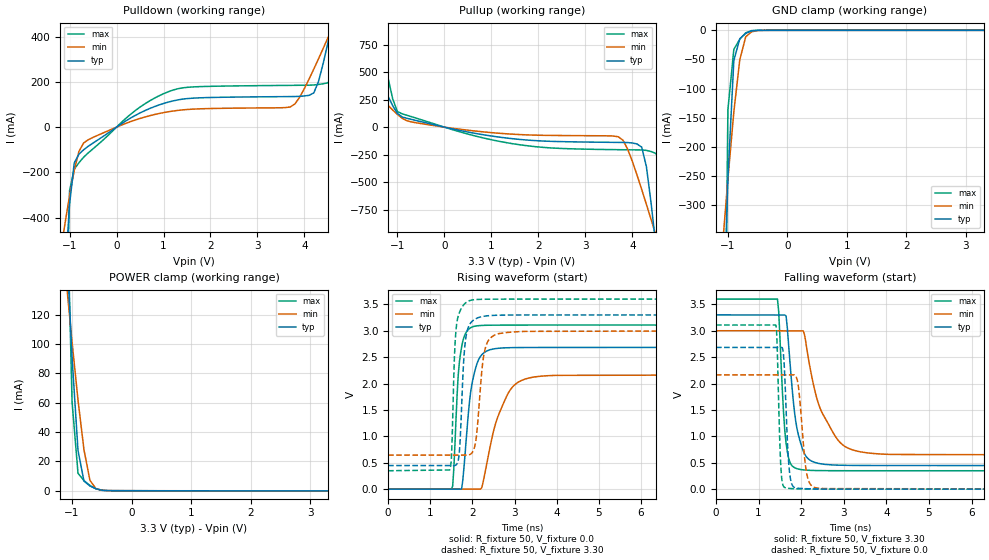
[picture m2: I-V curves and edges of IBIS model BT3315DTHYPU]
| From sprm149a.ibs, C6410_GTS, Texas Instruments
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[Model]   BT3315DTHYPU
Model_type   I/O
Vinh = 2.00
Vinl = 0.80
Enable   Active-Low
Polarity   Non-Inverting
| signals   A, GZ, Y
Vmeas = 1.5
|   typ   min   max
C_comp   1.5797p   1.5046p   1.7659p
|   typ   min   max
[Temperature Range]   25   -40   125
|   typ   min   max
[Voltage Range]   3.30V   3.00V   3.60V
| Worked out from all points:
|   slope of the pulldown table from 0 to 0.495 V, typ, clamps not added: 7.97 ohm
|   slope of the pullup table from 0 to 0.495 V, typ, clamps not added: 11.2 ohm
|   GND clamp passes 1 mA (typ) near -0.60 V on its own axis
|   POWER clamp passes 1 mA (typ) near -0.56 V on its own axis
|   rising waveform, R_fixture 50, V_fixture 0.0: 20-80 % time 218ps typ, 467ps min, 132ps max; typ from 0 V to 2.68 V
|   falling waveform, R_fixture 50, V_fixture 3.30: 20-80 % time 233ps typ, 559ps min, 132ps max; typ from 3.3 V to 0.447 V
|   rising waveform, R_fixture 50, V_fixture 3.30: 20-80 % time 109ps typ, 160ps min, 84ps max; typ from 0.447 V to 3.3 V
|   falling waveform, R_fixture 50, V_fixture 0.0: 20-80 % time 89.1ps typ, 141ps min, 66.8ps max; typ from 2.68 V to 0 V
[Pulldown]
|   Voltage   I(typ)   I(min)   I(max)
-3.3V     -10.22A    -3.602A    -42.43A
-1.1V     -673.7mA   -429.5mA   -1.184A
-1V       -341.4mA   -303.5mA   -280.7mA
-900mV    -157.9mA   -190.6mA   -185.8mA
-700mV    -99.92mA   -69.87mA   -132.7mA
1V        104.4mA    64.1mA     147.5mA
3.7V      134.9mA    89.21mA    184.4mA
4.2V      151.2mA    256.7mA    186.1mA
4.6V      467.5mA    441.4mA    222.4mA
4.7V      565.3mA    488.7mA    365.1mA
4.8V      664.8mA    536.2mA    566.6mA
6.6V      2.526A     1.409A     4.88A
[GND_clamp]
|   Voltage   I(typ)   I(min)   I(max)
-3.3V     -10.12A    -3.53A     -42.32A
-1.1V     -596.6mA   -381.7mA   -1.087A
-1V       -255.3mA   -255.1mA   -136.6mA
-900mV    -51.68mA   -139.8mA   -32.56mA
-800mV    -14.45mA   -50.51mA   -15.18mA
-700mV    -5.109mA   -10.94mA   -4.27mA
-600mV    -965.7uA   -2.448mA   -468.2uA
-400mV    -4.855uA   -52.49uA   -479.3nA
3.3V      133.2pA    4.204uA    266.4pA
[Pullup]
|   Voltage   I(typ)   I(min)   I(max)
-3.3V     2.416A     1.192A     5.478A
-2.7V     1.794A     902.2mA    4.011A
-1.9V     970.8mA    520mA      2.071A
-1.4V     469.5mA    286.9mA    889.2mA
-1.1V     193.7mA    154.9mA    254.5mA
-800mV    80.45mA    58.03mA    108mA
3.7V      -138.7mA   -87.59mA   -205mA
4.2V      -182.2mA   -567.8mA   -207.6mA
4.5V      -1.077A    -980.2mA   -239mA
4.6V      -1.482A    -1.121A    -323.2mA
4.7V      -1.898A    -1.262A    -1.22A
6.6V      -10.21A    -4.022A    -36.67A
[POWER_clamp]
|   Voltage   I(typ)   I(min)   I(max)
-3.3V     2.412A     1.185A     5.476A
-1.1V     175mA      143.9mA    225.4mA
-1V       90.98mA    101.4mA    60.69mA
-900mV    27.38mA    61.78mA    11.91mA
-800mV    6.568mA    27.98mA    6.904mA
-700mV    3.22mA     7.12mA     3.606mA
-600mV    1.379mA    1.452mA    1.304mA
-500mV    357.9uA    341.4uA    241uA
-400mV    65.66uA    67.61uA    56.94uA
3.3V      -108.4uA   -68.36uA   -162.2uA
[Ramp]
|   I(typ)   I(min)   I(max)
dV/dt_r   1.611/0.217n   1.299/0.467n   1.865/0.131n
dV/dt_f   1.712/0.233n   1.413/0.560n   1.951/0.131n
[Rising Waveform]
R_fixture = 50
V_fixture = 0.0
|  pu_on
|  TIME   V(typ)   V(min)   V(max)
0s        1nV        11nV       1nV
1.505ns   864.5uV    126.8uV    822.7pV
1.558ns   864.5uV    209.4uV    374.3mV
1.691ns   864.5uV    485.9uV    2.401V
1.771ns   155.3mV    935.9uV    2.796V
2.009ns   2.069V     946.2uV    3.076V
2.221ns   2.543V     27.12mV    3.1V
2.804ns   2.677V     1.745V     3.107V
3.229ns   2.682V     2.079V     3.107V
10ns      2.684V     2.164V     3.108V
[Falling Waveform]
R_fixture = 50
V_fixture = 3.30
V_fixture_min = 3.00
V_fixture_max = 3.60
|  pd_on
|  TIME   V(typ)   V(min)   V(max)
0s        3.3V       3V         3.6V
1.443ns   3.298V     3V         3.6V
1.587ns   3.298V     2.999V     1.432V
1.645ns   3.281V     2.998V     874.3mV
1.875ns   1.268V     2.998V     395.9mV
2.048ns   724.6mV    2.998V     365mV
2.192ns   557.6mV    2.37V      356.8mV
2.48ns    477.5mV    1.465V     351.5mV
3.172ns   450.4mV    753.8mV    349.2mV
10ns      447.4mV    645.6mV    348.8mV
[Rising Waveform]
R_fixture = 50
V_fixture = 3.30
V_fixture_min = 3.00
V_fixture_max = 3.60
|  pd_off
|  TIME   V(typ)   V(min)   V(max)
0s        447.4mV    645.6mV    348.8mV
1.462ns   447.4mV    646mV      363.7mV
1.629ns   472.6mV    646mV      3.141V
1.703ns   833.8mV    646mV      3.367V
1.815ns   2.663V     646mV      3.509V
1.926ns   3.106V     651.1mV    3.567V
2.075ns   3.224V     881.7mV    3.59V
2.298ns   3.277V     2.642V     3.596V
2.577ns   3.293V     2.934V     3.598V
10ns      3.3V       3V         3.6V
[Falling Waveform]
R_fixture = 50
V_fixture = 0.0
|  pu_off
|  TIME   V(typ)   V(min)   V(max)
0s        2.684V     2.164V     3.108V
1.409ns   2.683V     2.164V     3.102V
1.518ns   2.683V     2.163V     489.9mV
1.626ns   1.916V     2.163V     27.26mV
1.694ns   644.4mV    2.163V     16.96mV
1.762ns   141.7mV    2.163V     11.22mV
1.911ns   18.02mV    2.056V     5.662mV
2.115ns   8.749mV    366.9mV    2.601mV
2.318ns   4.71mV     31.81mV    1.445mV
10ns      258.9nV    3.87uV     130.5nV
